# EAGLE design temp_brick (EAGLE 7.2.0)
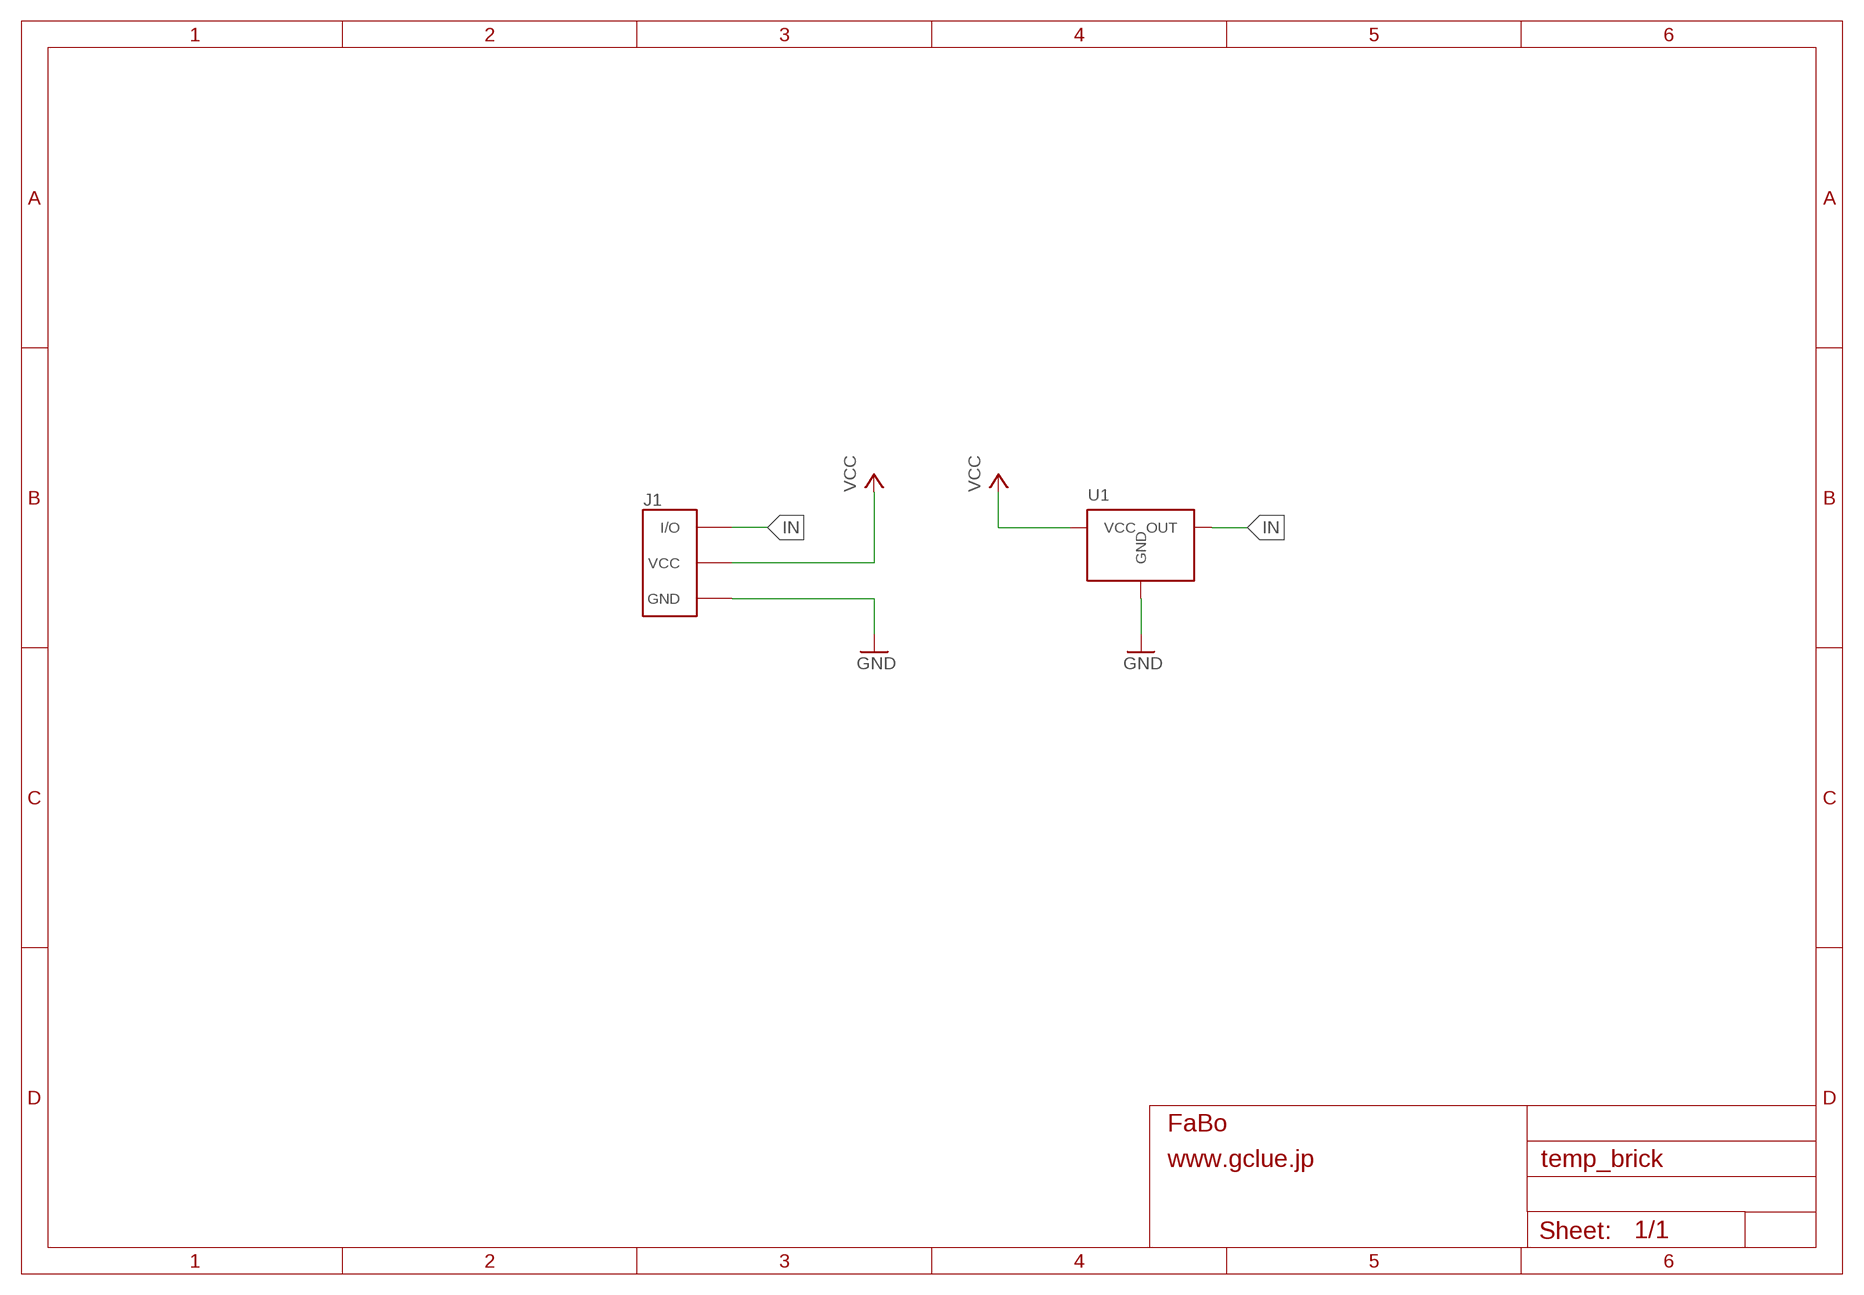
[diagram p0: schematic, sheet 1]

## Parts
J1  BRICK_3PIN  [BRICK_3PIN]
U1  SENSOR-LM60-TO92  [SENSOR-LM60-TO-92]

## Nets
GND: J1.GND U1.GND
IN: J1.IN/OUT(I/O) U1.OUT
VCC: J1.VCC U1.VCC

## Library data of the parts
J1 = Gclue:BRICK_3PIN: FaBo Brick 3pin
U1 = Gclue:SENSOR-LM60-: LM60 Temperature Sensor

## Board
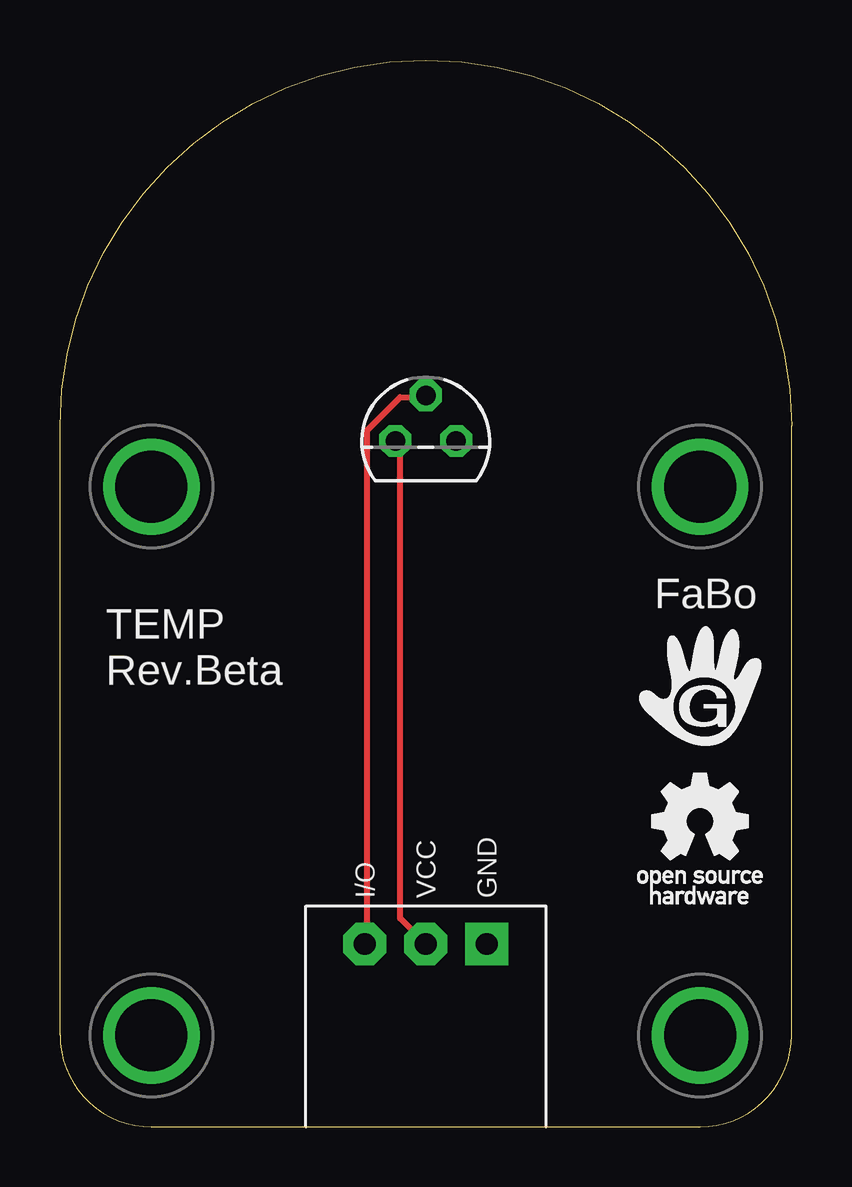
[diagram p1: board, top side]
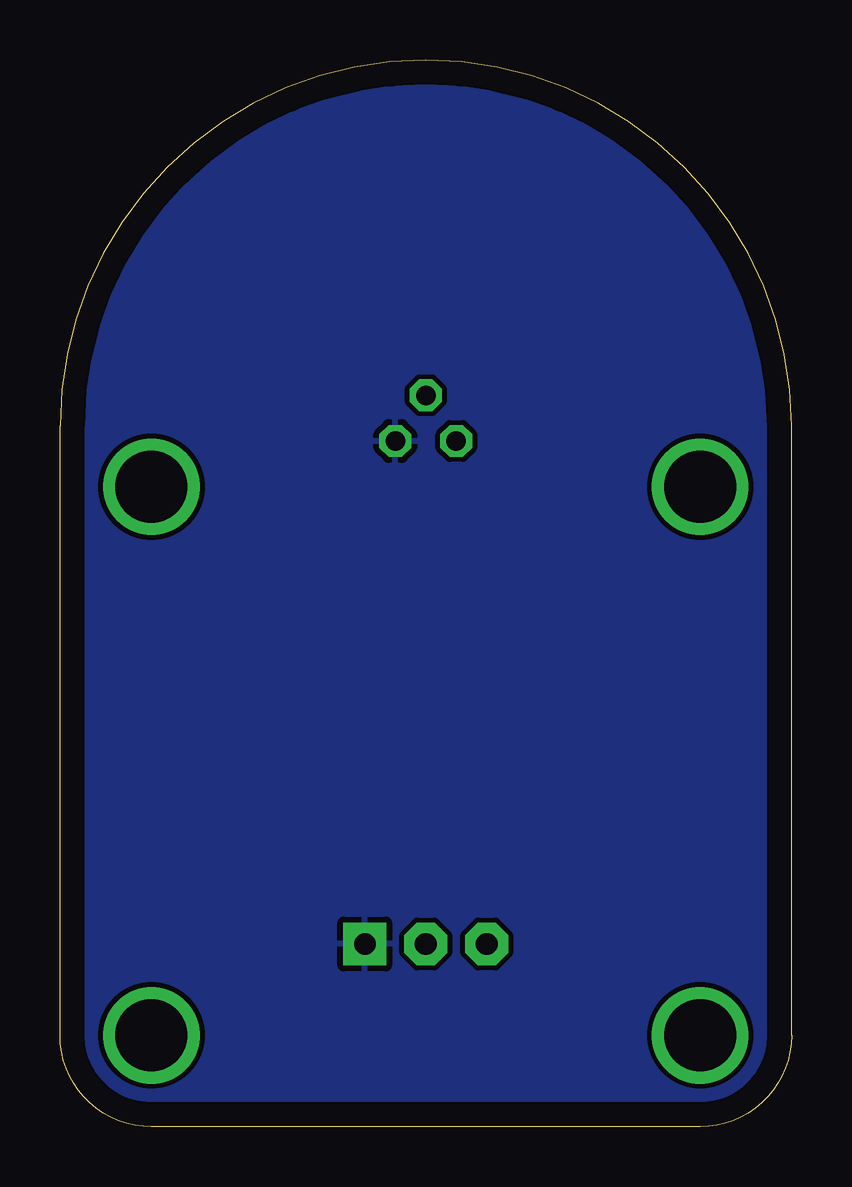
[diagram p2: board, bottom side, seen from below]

Size 30.48 x 44.45 mm. Coordinates in mm from the lower left corner, seen from the top.
Copper layers (1*16): Top 0.035mm / dielectric 1.5mm / Bottom 0.035mm
Design rules "default": minimum track width 10mil, minimum drill 24mil, track to track 8mil, track to pad 8mil, pad to pad 8mil, via to via 8mil, smd to smd 8mil, copper to edge 40mil, drill to drill 8mil, minimum pad ring 10mil, minimum via ring 8mil, stop-mask expansion 4mil, vias tented up to drill 0mil, thermal gap 10mil

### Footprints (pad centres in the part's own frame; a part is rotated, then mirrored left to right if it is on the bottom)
BRICK_3PIN = drill 0.9 pad 1.778 square: GND 2.54,-11.43 | drill 0.9 pad 1.778 octagon: IN/OUT -2.54,-11.43; VCC 0,-11.43 | drill 3 pad 3.81: P$1 -11.43,7.62; P$2 11.43,7.62; P$3 11.43,-15.24; P$4 -11.43,-15.24
SENSOR-LM60-TO-92 = drill 0.813 pad 1.27 octagon: GND 1.27,0; OUT 0,1.905; VCC -1.27,0

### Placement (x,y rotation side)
J1  15.24,19.05 0 top
U1  15.24,28.57 0 top
U$2  [LOGO_GCLUE_M]  26.67,18.41 0 top
U$3  [LOGO_OSHW_T_M]  26.67,12.7 0 top

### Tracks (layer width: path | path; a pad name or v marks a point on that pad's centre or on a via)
GND
  pour Bottom: 0,0 30.48,0 30.48,44.45 0,44.45
IN
  Top 0.254: U1.OUT 15.09,30.4 14.17,30.4 12.8,29.03 12.8,7.77 J1.IN/OUT
VCC
  Top 0.254: J1.VCC 14.17,8.69 14.17,28.57 U1.VCC

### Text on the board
tPlace: FaBo | TEMP / Rev.Beta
